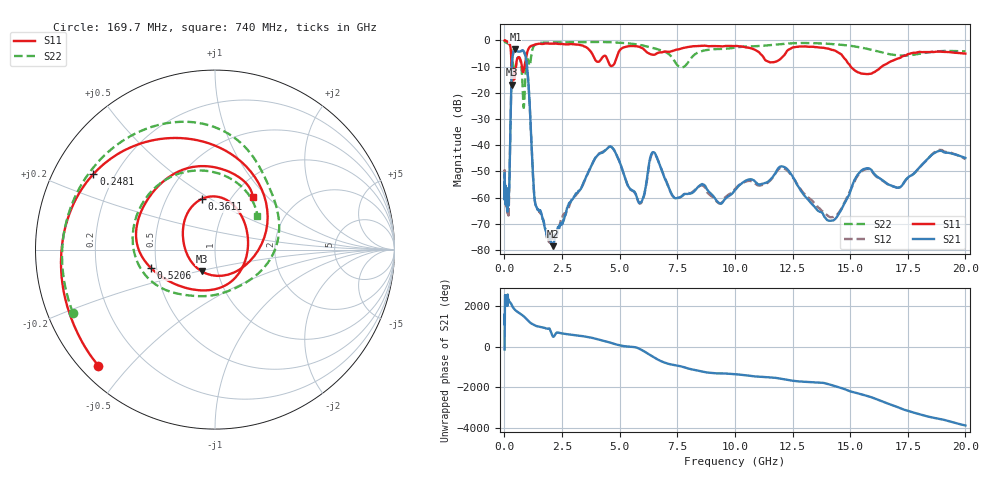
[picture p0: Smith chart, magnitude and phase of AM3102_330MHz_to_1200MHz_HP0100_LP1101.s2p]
! Date/Time: Tue, Sep 11, 2018 5:13 PM
! Network Analyzer: Agilent Technologies E8362B Rev: A.07.50.63
! Sweep from 0.010 to 20.000 GHz, 1601 Points, Sweep Type: LOG
! Power Supply: 4.949 V, 0.001 A
# Hz S DB R 50
!freq MagS11 AngS11 MagS21 AngS21 MagS12 AngS12 MagS22 AngS22
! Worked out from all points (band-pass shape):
!   1601 points, 10 MHz to 20 GHz, reference 50 ohm
!   highest |S21| = -3.42 dB at 478 MHz (marker M1); lowest = -78.6 dB at 2.124 GHz (marker M2)
!   |S21| within 3 dB of the highest: 351.6 MHz to 925.6 MHz (574 MHz wide, 89.9 % of centre)
!   lowest |S11| = -17.0 dB at 330 MHz (marker M3), VSWR 1.33, Z = 41.9 - j10.3 ohm
!   |S11| at or under -10 dB: 307.9 MHz to 503.8 MHz (195.9 MHz wide, 48.3 % of centre); 760.3 MHz to 868.8 MHz (108.4 MHz wide, 13.3 % of centre); 15.03 GHz to 16.37 GHz (1.348 GHz wide, 8.58 % of centre)
!   |S22| runs from -25.7 to -0.3 dB; largest |S21 - S12| = 0.012
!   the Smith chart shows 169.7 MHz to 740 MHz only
!   S11 on the Smith chart (normalised r, x): 169.7 MHz: 0.05, -0.41; 248.1 MHz: 0.12, +0.28; 361.1 MHz: 0.74, +0.46; 520.6 MHz: 0.46, -0.11; 740 MHz: 1.23, +0.83
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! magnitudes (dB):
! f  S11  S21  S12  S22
! 10 MHz  0.0  -50.7  -52.7  -0.3
! 35.55 MHz  0.0  -59.8  -59.9  -0.6
! 126.4 MHz  -0.4  -63.1  -64.0  -1.1
! 169.7 MHz  -0.8  -62.8  -66.0  -1.2
! 248.1 MHz  -2.0  -40.1  -40.1  -1.8
! 330 MHz  -17.0  -8.8  -8.8  -5.8
! 361.1 MHz  -10.7  -5.8  -5.9  -8.1
! 447.2 MHz  -14.0  -3.5  -3.5  -11.9
! 478 MHz  -12.3  -3.4  -3.4  -10.7
! 520.6 MHz  -8.6  -3.7  -3.8  -8.3
! 740 MHz  -8.8  -4.0  -4.0  -10.4
! 837.2 MHz  -11.6  -4.1  -4.2  -25.7
! 984 MHz  -4.8  -10.1  -10.1  -7.6
! 1.309 GHz  -1.6  -60.5  -60.3  -1.8
! 1.59 GHz  -1.3  -65.8  -66.2  -0.9
! 2.124 GHz  -1.2  -78.6  -74.9  -0.7
! 4.5 GHz  -8.0  -41.0  -40.9  -0.6
! 5.652 GHz  -2.2  -57.9  -58.2  -1.4
! 6.487 GHz  -5.5  -42.7  -43.1  -3.0
! 12.09 GHz  -6.1  -48.2  -48.7  -1.3
! 14.07 GHz  -3.2  -68.8  -67.3  -1.3
! 20 GHz  -5.0  -44.9  -45.3  -4.2
